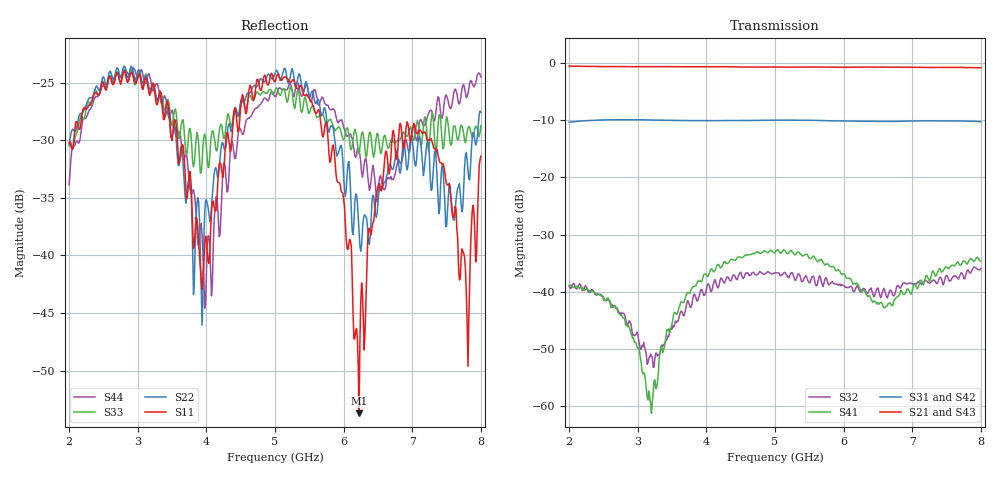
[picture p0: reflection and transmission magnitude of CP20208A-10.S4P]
! Amtery
! Email: info@amtery.com
! Phone: 886-2-2883-7839
! Model Number: CP20208A-10
! 4-port S-parameter measurement data for Bi-Directional Coupler
! Frequency Range: 2 GHz to 8 GHz
! Port 1: Input
! Port 2: Output
! Port 3: Coupled Forward
! Port 4: Coupled Reverse
# Hz S dB R 50
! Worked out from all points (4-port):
!   481 points, 2 GHz to 8 GHz, reference 50 ohm
!   strongest paths, dB at 2 GHz, 3.5 GHz, 5 GHz, 6.5 GHz, 8 GHz:
!     S21: -0.6, -0.7, -0.7, -0.7, -0.9
!     S43: -0.6, -0.7, -0.8, -0.9, -0.9
!     S31: -10.4, -10.1, -10.0, -10.2, -10.3
!     S42: -10.4, -10.2, -10.2, -10.5, -10.5
!     S41: -38.9, -45.6, -33.2, -41.9, -34.6
!     S32: -39.0, -46.5, -36.7, -39.3, -35.9
!   lowest |S11| = -53.7 dB at 6.225 GHz (marker M1), VSWR 1.00, Z = 49.8 - j0.00754 ohm
!   |S11| at or under -10 dB: start of sweep to end of sweep
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2e9  -30.21 41.7  -0.60 126.5  -10.37 -94.1  -39.01 179.5
     -0.59 126.5  -30.32 -0.1  -38.90 161.6  -10.45 175.7
     -10.37 -94.1  -38.96 159.7  -30.51 15.8  -0.61 135.0
     -38.86 -179.5  -10.45 175.8  -0.61 135.2  -33.86 35.7
3.0625e9  -25.34 -79.9  -0.69 4.6  -9.97 -177.5  -52.75 14.2
          -0.67 4.7  -25.01 -85.4  -51.58 8.2  -10.12 20.4
          -9.96 -177.4  -49.37 7.6  -25.50 -86.2  -0.73 17.9
          -53.96 17.0  -10.11 20.4  -0.72 18.1  -23.95 -53.7
4.0125e9  -39.47 -65.9  -0.71 -105.1  -10.11 116.4  -37.38 -12.6
          -0.70 -105.0  -35.49 -57.3  -39.20 -55.1  -10.32 -129.0
          -10.10 116.4  -38.90 -57.3  -31.57 -97.4  -0.75 -87.8
          -37.32 -9.5  -10.32 -128.8  -0.75 -87.5  -39.04 96.9
4.95e9  -24.17 -120.2  -0.75 146.8  -10.04 52.6  -32.79 -174.2
        -0.74 147.0  -24.63 -114.9  -36.46 144.7  -10.23 83.0
        -10.03 52.6  -36.82 146.3  -25.75 -149.1  -0.81 168.6
        -32.85 -171.0  -10.24 83.3  -0.81 168.9  -25.78 -52.5
6.225e9  -53.71 -177.9  -0.78 -0.0  -10.22 -35.0  -39.94 -13.3
         -0.76 0.1  -37.82 -171.9  -38.87 -35.4  -10.51 -117.7
         -10.21 -34.9  -39.62 -41.2  -31.16 145.6  -0.88 27.0
         -39.10 -12.0  -10.51 -117.4  -0.85 27.5  -30.72 137.1
7.05e9  -29.11 -170.1  -0.79 -95.2  -10.17 -91.4  -39.16 -69.6
        -0.79 -95.4  -32.24 179.7  -38.36 -140.7  -10.41 112.0
        -10.16 -91.7  -38.59 -135.4  -29.00 103.7  -0.85 -64.4
        -38.83 -72.0  -10.42 112.5  -0.86 -63.9  -29.77 -44.4
8e9  -31.38 -120.0  -0.86 155.5  -10.32 -163.4  -34.25 146.3
     -0.86 155.5  -27.55 -152.2  -34.79 83.3  -10.56 -28.9
     -10.31 -163.9  -35.92 88.4  -28.71 -25.5  -0.96 -169.2
     -34.64 144.9  -10.54 -29.0  -0.94 -168.8  -24.50 -133.7
